| IBIS file stm32h523_533_lqfp48.ibs
[IBIS ver] 4.2
[File name] stm32h523_533_lqfp48.ibs
[File Rev] 0.2
[Date] 07-05-2024
[Source] Data Created at STMicroelectronics
[Notes]  File originated from ELDO simulations.
[Disclaimer]  This information is for modeling purpose only and is
   not guaranteed. The information is subject to change without
   notice.
[Copyright] Copyright 2024 STMicroelectronics Inc.
|   Component stm32h523_533_lqfp48
[Component] stm32h523_533_lqfp48
[Manufacturer] STMicroelectronics
[Package]
| variable   typ   min   max
R_pkg  0  NA  NA
L_pkg  0  NA  NA
C_pkg  0  NA  NA
[Pin]   signal_name   model_name
1  VBAT  power
2  PC13  io8_ft_i3c_spi_v33
3  PC14-OSC32_IN  io_ft_tamp
4  PC15-OSC32_OUT  io_ft_tamp
5  PH0-OSC_IN  io8_ft_i3c_spi
6  PH1-OSC_OUT  io8_ft_i3c_spi
7  NRST  ioreset_ft_v33
8  VSSA  nc
9  VDDA  nc
10  PA0  io8_ft_spi
11  PA1  io8_ft_spi_tamp
12  PA2  io8_ft_spi
13  PA3  io8_ft_spi
14  PA4  io8_ft_spi
15  PA5  io8_ft_spi
16  PA6  io8_ft_spi
17  PA7  io8_ft_spi
18  PB0  io8_ft_spi
19  PB1  io8_ft_spi
20  PB2  io8_ft_i3c_spi
21  PB10  io8_ft_i3c_spi
22  VCAP  nc
23  VSS  gnd
24  VDD  power
25  PB12  io8_ft_i3c_spi
26  PB13  nc
27  PB14  nc
28  PB15  io8_ft_spi
29  PA8  io8_ft_i3c_spi
30  PA9  io8_ft_i3c_spi
31  PA10  io8_ft_i3c_spi
32  PA11  io8usb_ft_i3c_spi_phy
33  PA12  io8usb_ft_i3c_spi_phy
34  PA13  io8_ft_i3c_spi
35  VSS  gnd
36  VDD  power
37  PA14  io8_ft_i3c_spi
38  PA15  io8_ft_i3c_spi
39  PB3  io8_ft_i3c_spi
40  PB4  io8_ft_i3c_spi
41  PB5  io8_ft_i3c_spi
42  PB6  io8_ft_i3c_spi
43  PB7  io8_ft_i3c_spi
44  BOOT0  vpphv
45  PB8  io8_ft_i3c_spi
46  VCAP  nc
47  VSS  gnd
48  VDD  power
[Package Model]   478-lqfp-7x7-48-240315
[Pin Mapping]   pulldown_ref   pullup_ref   | Comment
1  nc  vsw
2  gndio  vddio  | Depending on IO usage
| 2  gndio  vsw  | Depending on IO usage
3  gndio  vddio  | Depending on IO usage
| 3  gndio  vsw  | Depending on IO usage
4  gndio  vddio  | Depending on IO usage
| 4  gndio  vsw  | Depending on IO usage
5  gndio  vddio
6  gndio  vddio
7  gndio  vddio
8  nc  nc
9  nc  nc
10  gndio  vddio
11  gndio  vddio
12  gndio  vddio
13  gndio  vddio
14  gndio  vddio
15  gndio  vddio
16  gndio  vddio
17  gndio  vddio
18  gndio  vddio
19  gndio  vddio
20  gndio  vddio
21  gndio  vddio
22  nc  nc
23  gndio  nc
24  nc  vddio
25  gndio  vddio
26  nc  nc
27  nc  nc
28  gndio  vddio
29  gndio  vddio
30  gndio  vddio
31  gndio  vddio
32  gndio  vddusb  | Depending on IO usage
| 32  gndio  vddio  | Depending on IO usage
33  gndio  vddusb  | Depending on IO usage
| 33  gndio  vddio  | Depending on IO usage
34  gndio  vddio
35  gndio  nc
36  nc  vddusb
37  gndio  vddio
38  gndio  vddio
39  gndio  vddio
40  gndio  vddio
41  gndio  vddio
42  gndio  vddio
43  gndio  vddio
44  gndio  vddio
45  gndio  vddio
46  nc  nc
47  gndio  nc
48  nc  vddio
|[Diff Pin]  inv_pin  vdiff  tdelay_typ  tdelay_min  tdelay_max
|33  32  NA  NA  NA  NA
[Model Selector] io8_ft_i3c_spi
io8_ft_spi_ls_1v2 "GPIO SPI - 5V tolerant - low speed - 1.2V range"
io8_ft_spi_ls_1v8 "GPIO SPI - 5V tolerant - low speed - 1.8V range"
io8_ft_spi_ls_3v3 "GPIO SPI - 5V tolerant - low speed - 3.3V range"
io8_ft_spi_ms_1v2 "GPIO SPI - 5V tolerant - med speed - 1.2V range"
io8_ft_spi_ms_1v8 "GPIO SPI - 5V tolerant - med speed - 1.8V range"
io8_ft_spi_ms_3v3 "GPIO SPI - 5V tolerant - med speed - 3.3V range"
io8_ft_spi_fs_1v2 "GPIO SPI - 5V tolerant - fast speed - 1.2V range"
io8_ft_spi_fs_1v8 "GPIO SPI - 5V tolerant - fast speed - 1.8V range"
io8_ft_spi_fs_3v3 "GPIO SPI - 5V tolerant - fast speed - 3.3V range"
io8_ft_spi_hs_1v2 "GPIO SPI - 5V tolerant - high speed - 1.2V range"
io8_ft_spi_hs_1v8 "GPIO SPI - 5V tolerant - high speed - 1.8V range"
io8_ft_spi_hs_3v3 "GPIO SPI - 5V tolerant - high speed - 3.3V range"
io8_ft_hslv_spi_ls_1v2 "GPIO SPI low volt opt - 5V tolerant - low speed - 1.2V range"
io8_ft_hslv_spi_ls_1v8 "GPIO SPI low volt opt - 5V tolerant - low speed - 1.8V range"
io8_ft_hslv_spi_ls_2v5 "GPIO SPI low volt opt - 5V tolerant - low speed - 2.5V range"
io8_ft_hslv_spi_ms_1v2 "GPIO SPI low volt opt - 5V tolerant - med speed - 1.2V range"
io8_ft_hslv_spi_ms_1v8 "GPIO SPI low volt opt - 5V tolerant - med speed - 1.8V range"
io8_ft_hslv_spi_ms_2v5 "GPIO SPI low volt opt - 5V tolerant - med speed - 2.5V range"
io8_ft_hslv_spi_fs_1v2 "GPIO SPI low volt opt - 5V tolerant - fast speed - 1.2V range"
io8_ft_hslv_spi_fs_1v8 "GPIO SPI low volt opt - 5V tolerant - fast speed - 1.8V range"
io8_ft_hslv_spi_fs_2v5 "GPIO SPI low volt opt - 5V tolerant - fast speed - 2.5V range"
io8_ft_hslv_spi_hs_1v2 "GPIO SPI low volt opt - 5V tolerant - high speed - 1.2V range"
io8_ft_hslv_spi_hs_1v8 "GPIO SPI low volt opt - 5V tolerant - high speed - 1.8V range"
io8_ft_hslv_spi_hs_2v5 "GPIO SPI low volt opt - 5V tolerant - high speed - 2.5V range"
io8_ft_i3c_spi_ls_1v2 "GPIO SPI with I3C open-drain - 5V tolerant - low speed - 1.2V range"
io8_ft_i3c_spi_ls_1v8 "GPIO SPI with I3C open-drain - 5V tolerant - low speed - 1.8V range"
io8_ft_i3c_spi_ls_3v3 "GPIO SPI with I3C open-drain - 5V tolerant - low speed - 3.3V range"
io8_ft_i3c_spi_ms_1v2 "GPIO SPI with I3C open-drain - 5V tolerant - med speed - 1.2V range"
io8_ft_i3c_spi_ms_1v8 "GPIO SPI with I3C open-drain - 5V tolerant - med speed - 1.8V range"
io8_ft_i3c_spi_ms_3v3 "GPIO SPI with I3C open-drain - 5V tolerant - med speed - 3.3V range"
io8_ft_i3c_spi_fs_1v2 "GPIO SPI with I3C open-drain - 5V tolerant - fast speed - 1.2V range"
io8_ft_i3c_spi_fs_1v8 "GPIO SPI with I3C open-drain - 5V tolerant - fast speed - 1.8V range"
io8_ft_i3c_spi_fs_3v3 "GPIO SPI with I3C open-drain - 5V tolerant - fast speed - 3.3V range"
io8_ft_i3c_spi_hs_1v2 "GPIO SPI with I3C open-drain - 5V tolerant - high speed - 1.2V range"
io8_ft_i3c_spi_hs_1v8 "GPIO SPI with I3C open-drain - 5V tolerant - high speed - 1.8V range"
io8_ft_i3c_spi_hs_3v3 "GPIO SPI with I3C open-drain - 5V tolerant - high speed - 3.3V range"
io8_ft_hslv_i3c_spi_ls_1v2 "GPIO SPI low volt opt with I3C open-drain - 5V tolerant - low speed - 1.2V range"
io8_ft_hslv_i3c_spi_ls_1v8 "GPIO SPI low volt opt with I3C open-drain - 5V tolerant - low speed - 1.8V range"
io8_ft_hslv_i3c_spi_ls_2v5 "GPIO SPI low volt opt with I3C open-drain - 5V tolerant - low speed - 2.5V range"
io8_ft_hslv_i3c_spi_ms_1v2 "GPIO SPI low volt opt with I3C open-drain - 5V tolerant - med speed - 1.2V range"
io8_ft_hslv_i3c_spi_ms_1v8 "GPIO SPI low volt opt with I3C open-drain - 5V tolerant - med speed - 1.8V range"
io8_ft_hslv_i3c_spi_ms_2v5 "GPIO SPI low volt opt with I3C open-drain - 5V tolerant - med speed - 2.5V range"
io8_ft_hslv_i3c_spi_fs_1v2 "GPIO SPI low volt opt with I3C open-drain - 5V tolerant - fast speed - 1.2V range"
io8_ft_hslv_i3c_spi_fs_1v8 "GPIO SPI low volt opt with I3C open-drain - 5V tolerant - fast speed - 1.8V range"
io8_ft_hslv_i3c_spi_fs_2v5 "GPIO SPI low volt opt with I3C open-drain - 5V tolerant - fast speed - 2.5V range"
io8_ft_hslv_i3c_spi_hs_1v2 "GPIO SPI low volt opt with I3C open-drain - 5V tolerant - high speed - 1.2V range"
io8_ft_hslv_i3c_spi_hs_1v8 "GPIO SPI low volt opt with I3C open-drain - 5V tolerant - high speed - 1.8V range"
io8_ft_hslv_i3c_spi_hs_2v5 "GPIO SPI low volt opt with I3C open-drain - 5V tolerant - high speed - 2.5V range"
io8_ft_i3c_fmp_spi_3v3 "GPIO SPI with I3C fm+ open-drain - 5V tolerant - 3.3V range"
io8_ft_i3c_fmp_spi_1v8 "GPIO SPI with I3C fm+ open-drain - 5V tolerant - 1.8V range"
io8_ft_i3c_fmp_spi_1v2 "GPIO SPI with I3C fm+ open-drain - 5V tolerant - 1.2V range"
[Model Selector] io8_ft_i3c_spi_v33
io8_ft_spi_v33_ls_1v2 ""GPIO SPI V33 - 5V tolerant - low speed - 1.2V range"
io8_ft_spi_v33_ls_1v8 ""GPIO SPI V33 - 5V tolerant - low speed - 1.8V range"
io8_ft_spi_v33_ls_3v3 ""GPIO SPI V33 - 5V tolerant - low speed - 3.3V range"
io8_ft_spi_v33_ms_1v2 ""GPIO SPI V33 - 5V tolerant - med speed - 1.2V range"
io8_ft_spi_v33_ms_1v8 ""GPIO SPI V33 - 5V tolerant - med speed - 1.8V range"
io8_ft_spi_v33_ms_3v3 ""GPIO SPI V33 - 5V tolerant - med speed - 3.3V range"
io8_ft_spi_v33_fs_1v2 ""GPIO SPI V33 - 5V tolerant - fast speed - 1.2V range
io8_ft_spi_v33_fs_1v8 ""GPIO SPI V33 - 5V tolerant - fast speed - 1.8V range
io8_ft_spi_v33_fs_3v3 ""GPIO SPI V33 - 5V tolerant - fast speed - 3.3V range
io8_ft_spi_v33_hs_1v2 ""GPIO SPI V33 - 5V tolerant - high speed - 1.2V range
io8_ft_spi_v33_hs_1v8 ""GPIO SPI V33 - 5V tolerant - high speed - 1.8V range
io8_ft_spi_v33_hs_3v3 ""GPIO SPI V33 - 5V tolerant - high speed - 3.3V range
io8_ft_hslv_spi_v33_ls_1v2 "GPIO SPI V33 low volt opt - 5V tolerant - low speed - 1.2V range""
io8_ft_hslv_spi_v33_ls_1v8 "GPIO SPI V33 low volt opt - 5V tolerant - low speed - 1.8V range""
io8_ft_hslv_spi_v33_ls_2v5 "GPIO SPI V33 low volt opt - 5V tolerant - low speed - 2.5V range""
io8_ft_hslv_spi_v33_ms_1v2 "GPIO SPI V33 low volt opt - 5V tolerant - med speed - 1.2V range""
io8_ft_hslv_spi_v33_ms_1v8 "GPIO SPI V33 low volt opt - 5V tolerant - med speed - 1.8V range""
io8_ft_hslv_spi_v33_ms_2v5 "GPIO SPI V33 low volt opt - 5V tolerant - med speed - 2.5V range""
io8_ft_hslv_spi_v33_fs_1v2 "GPIO SPI V33 low volt opt - 5V tolerant - fast speed - 1.2V range"
io8_ft_hslv_spi_v33_fs_1v8 "GPIO SPI V33 low volt opt - 5V tolerant - fast speed - 1.8V range"
io8_ft_hslv_spi_v33_fs_2v5 "GPIO SPI V33 low volt opt - 5V tolerant - fast speed - 2.5V range"
io8_ft_hslv_spi_v33_hs_1v2 "GPIO SPI V33 low volt opt - 5V tolerant - high speed - 1.2V range"
io8_ft_hslv_spi_v33_hs_1v8 "GPIO SPI V33 low volt opt - 5V tolerant - high speed - 1.8V range"
io8_ft_hslv_spi_v33_hs_2v5 "GPIO SPI V33 low volt opt - 5V tolerant - high speed - 2.5V range"
io8_ft_i3c_spi_v33_ls_1v2 "GPIO SPI V33 with I3C open-drain - 5V tolerant - low speed - 1.2V range"
io8_ft_i3c_spi_v33_ls_1v8 "GPIO SPI V33 with I3C open-drain - 5V tolerant - low speed - 1.8V range"
io8_ft_i3c_spi_v33_ls_3v3 "GPIO SPI V33 with I3C open-drain - 5V tolerant - low speed - 3.3V range"
io8_ft_i3c_spi_v33_ms_1v2 "GPIO SPI V33 with I3C open-drain - 5V tolerant - med speed - 1.2V range"
io8_ft_i3c_spi_v33_ms_1v8 "GPIO SPI V33 with I3C open-drain - 5V tolerant - med speed - 1.8V range"
io8_ft_i3c_spi_v33_ms_3v3 "GPIO SPI V33 with I3C open-drain - 5V tolerant - med speed - 3.3V range"
io8_ft_i3c_spi_v33_fs_1v2 "GPIO SPI V33 with I3C open-drain - 5V tolerant - fast speed - 1.2V range"
io8_ft_i3c_spi_v33_fs_1v8 "GPIO SPI V33 with I3C open-drain - 5V tolerant - fast speed - 1.8V range"
io8_ft_i3c_spi_v33_fs_3v3 "GPIO SPI V33 with I3C open-drain - 5V tolerant - fast speed - 3.3V range"
io8_ft_i3c_spi_v33_hs_1v2 "GPIO SPI V33 with I3C open-drain - 5V tolerant - high speed - 1.2V range"
io8_ft_i3c_spi_v33_hs_1v8 "GPIO SPI V33 with I3C open-drain - 5V tolerant - high speed - 1.8V range"
io8_ft_i3c_spi_v33_hs_3v3 "GPIO SPI V33 with I3C open-drain - 5V tolerant - high speed - 3.3V range"
io8_ft_hslv_i3c_spi_v33_ls_1v2 "GPIO SPI V33 low volt opt with I3C open-drain - 5V tolerant - low speed - 1.2V range"
io8_ft_hslv_i3c_spi_v33_ls_1v8 "GPIO SPI V33 low volt opt with I3C open-drain - 5V tolerant - low speed - 1.8V range"
io8_ft_hslv_i3c_spi_v33_ls_2v5 "GPIO SPI V33 low volt opt with I3C open-drain - 5V tolerant - low speed - 2.5V range"
io8_ft_hslv_i3c_spi_v33_ms_1v2 "GPIO SPI V33 low volt opt with I3C open-drain - 5V tolerant - med speed - 1.2V range"
io8_ft_hslv_i3c_spi_v33_ms_1v8 "GPIO SPI V33 low volt opt with I3C open-drain - 5V tolerant - med speed - 1.8V range"
io8_ft_hslv_i3c_spi_v33_ms_2v5 "GPIO SPI V33 low volt opt with I3C open-drain - 5V tolerant - med speed - 2.5V range"
io8_ft_hslv_i3c_spi_v33_fs_1v2 "GPIO SPI V33 low volt opt with I3C open-drain - 5V tolerant - fast speed - 1.2V range"
io8_ft_hslv_i3c_spi_v33_fs_1v8 "GPIO SPI V33 low volt opt with I3C open-drain - 5V tolerant - fast speed - 1.8V range"
io8_ft_hslv_i3c_spi_v33_fs_2v5 "GPIO SPI V33 low volt opt with I3C open-drain - 5V tolerant - fast speed - 2.5V range"
io8_ft_hslv_i3c_spi_v33_hs_1v2 "GPIO SPI V33 low volt opt with I3C open-drain - 5V tolerant - high speed - 1.2V range"
io8_ft_hslv_i3c_spi_v33_hs_1v8 "GPIO SPI V33 low volt opt with I3C open-drain - 5V tolerant - high speed - 1.8V range"
io8_ft_hslv_i3c_spi_v33_hs_2v5 "GPIO SPI V33 low volt opt with I3C open-drain - 5V tolerant - high speed - 2.5V range"
io8_ft_i3c_fmp_spi_v33_3v3 "GPIO SPI V33 with I3C fm+ open-drain - 5V tolerant - 3.3V range"
io8_ft_i3c_fmp_spi_v33_1v8 "GPIO SPI V33 with I3C fm+ open-drain - 5V tolerant - 1.8V range"
io8_ft_i3c_fmp_spi_v33_1v2 "GPIO SPI V33 with I3C fm+ open-drain - 5V tolerant - 1.2V range"
[Model Selector] io8_ft_spi
io8_ft_spi_ls_1v2 "GPIO SPI - 5V tolerant - low speed - 1.2V range"
io8_ft_spi_ls_1v8 "GPIO SPI - 5V tolerant - low speed - 1.8V range"
io8_ft_spi_ls_3v3 "GPIO SPI - 5V tolerant - low speed - 3.3V range"
io8_ft_spi_ms_1v2 "GPIO SPI- 5V tolerant - med speed - 1.2V range"
io8_ft_spi_ms_1v8 "GPIO SPI- 5V tolerant - med speed - 1.8V range"
io8_ft_spi_ms_3v3 "GPIO SPI- 5V tolerant - med speed - 3.3V range"
io8_ft_spi_fs_1v2 "GPIO SPI- 5V tolerant - fast speed - 1.2V range"
io8_ft_spi_fs_1v8 "GPIO SPI- 5V tolerant - fast speed - 1.8V range"
io8_ft_spi_fs_3v3 "GPIO SPI- 5V tolerant - fast speed - 3.3V range"
io8_ft_spi_hs_1v2 "GPIO SPI- 5V tolerant - high speed - 1.2V range"
io8_ft_spi_hs_1v8 "GPIO SPI- 5V tolerant - high speed - 1.8V range"
io8_ft_spi_hs_3v3 "GPIO SPI- 5V tolerant - high speed - 3.3V range"
io8_ft_hslv_spi_ls_1v2 "GPIO SPI low volt opt - 5V tolerant - low speed - 1.2V range"
io8_ft_hslv_spi_ls_1v8 "GPIO SPI low volt opt - 5V tolerant - low speed - 1.8V range"
io8_ft_hslv_spi_ls_2v5 "GPIO SPI low volt opt - 5V tolerant - low speed - 2.5V range"
io8_ft_hslv_spi_ms_1v2 "GPIO SPI low volt opt - 5V tolerant - med speed - 1.2V range"
io8_ft_hslv_spi_ms_1v8 "GPIO SPI low volt opt - 5V tolerant - med speed - 1.8V range"
io8_ft_hslv_spi_ms_2v5 "GPIO SPI low volt opt - 5V tolerant - med speed - 2.5V range"
io8_ft_hslv_spi_fs_1v2 "GPIO SPI low volt opt - 5V tolerant - fast speed - 1.2V range"
io8_ft_hslv_spi_fs_1v8 "GPIO SPI low volt opt - 5V tolerant - fast speed - 1.8V range"
io8_ft_hslv_spi_fs_2v5 "GPIO SPI low volt opt - 5V tolerant - fast speed - 2.5V range"
io8_ft_hslv_spi_hs_1v2 "GPIO SPI low volt opt - 5V tolerant - high speed - 1.2V range"
io8_ft_hslv_spi_hs_1v8 "GPIO SPI low volt opt - 5V tolerant - high speed - 1.8V range"
io8_ft_hslv_spi_hs_2v5 "GPIO SPI low volt opt - 5V tolerant - high speed - 2.5V range"
[Model Selector] io8_ft_spi_tamp
io8_ft_spi_ls_1v2 "GPIO SPI - 5V tolerant - low speed - 1.2V range"
io8_ft_spi_ls_1v8 "GPIO SPI - 5V tolerant - low speed - 1.8V range"
io8_ft_spi_ls_3v3 "GPIO SPI- 5V tolerant - low speed - 3.3V range"
io8_ft_spi_ms_1v2 "GPIO SPI - 5V tolerant - med speed - 1.2V range"
io8_ft_spi_ms_1v8 "GPIO SPI - 5V tolerant - med speed - 1.8V range"
io8_ft_spi_ms_3v3 "GPIO SPI - 5V tolerant - med speed - 3.3V range"
io8_ft_spi_fs_1v2 "GPIO SPI - 5V tolerant - fast speed - 1.2V range"
io8_ft_spi_fs_1v8 "GPIO SPI - 5V tolerant - fast speed - 1.8V range"
io8_ft_spi_fs_3v3 "GPIO SPI - 5V tolerant - fast speed - 3.3V range"
io8_ft_spi_hs_1v2 "GPIO SPI - 5V tolerant - high speed - 1.2V range"
io8_ft_spi_hs_1v8 "GPIO SPI - 5V tolerant - high speed - 1.8V range"
io8_ft_spi_hs_3v3 "GPIO SPI - 5V tolerant - high speed - 3.3V range"
io8_ft_hslv_spi_ls_1v2 "GPIO SPI low volt opt - 5V tolerant - low speed - 1.2V range"
io8_ft_hslv_spi_ls_1v8 "GPIO SPI low volt opt - 5V tolerant - low speed - 1.8V range"
io8_ft_hslv_spi_ls_2v5 "GPIO SPI low volt opt - 5V tolerant - low speed - 2.5V range"
io8_ft_hslv_spi_ms_1v2 "GPIO SPI low volt opt - 5V tolerant - med speed - 1.2V range"
io8_ft_hslv_spi_ms_1v8 "GPIO SPI low volt opt - 5V tolerant - med speed - 1.8V range"
io8_ft_hslv_spi_ms_2v5 "GPIO SPI low volt opt - 5V tolerant - med speed - 2.5V range"
io8_ft_hslv_spi_fs_1v2 "GPIO SPI low volt opt - 5V tolerant - fast speed - 1.2V range"
io8_ft_hslv_spi_fs_1v8 "GPIO SPI low volt opt - 5V tolerant - fast speed - 1.8V range"
io8_ft_hslv_spi_fs_2v5 "GPIO SPI low volt opt - 5V tolerant - fast speed - 2.5V range"
io8_ft_hslv_spi_hs_1v2 "GPIO SPI low volt opt - 5V tolerant - high speed - 1.2V range"
io8_ft_hslv_spi_hs_1v8 "GPIO SPI low volt opt - 5V tolerant - high speed - 1.8V range"
io8_ft_hslv_spi_hs_2v5 "GPIO SPI low volt opt - 5V tolerant - high speed - 2.5V range
io8_ft_tamp_v33_1v2 "IO tamper - 5V tolerant - 1.2V range"
io8_ft_tamp_v33_1v8 "IO tamper - 5V tolerant - 1.8V range"
io8_ft_tamp_v33_3v3 "IO tamper - 5V tolerant - 3.3V range"
[Model Selector] io8usb_ft_i3c_spi_phy
io8_ft_spi_ls_1v2 "GPIO SPI - 5V tolerant - low speed - 1.2V range"
io8_ft_spi_ls_1v8 "GPIO SPI - 5V tolerant - low speed - 1.8V range"
io8_ft_spi_ls_3v3 "GPIO SPI - 5V tolerant - low speed - 3.3V range"
io8_ft_spi_ms_1v2 "GPIO SPI - 5V tolerant - med speed - 1.2V range"
io8_ft_spi_ms_1v8 "GPIO SPI - 5V tolerant - med speed - 1.8V range"
io8_ft_spi_ms_3v3 "GPIO SPI - 5V tolerant - med speed - 3.3V range"
io8_ft_spi_fs_1v2 "GPIO SPI - 5V tolerant - fast speed - 1.2V range"
io8_ft_spi_fs_1v8 "GPIO SPI - 5V tolerant - fast speed - 1.8V range"
io8_ft_spi_fs_3v3 "GPIO SPI - 5V tolerant - fast speed - 3.3V range"
io8_ft_spi_hs_1v2 "GPIO SPI - 5V tolerant - high speed - 1.2V range"
io8_ft_spi_hs_1v8 "GPIO SPI - 5V tolerant - high speed - 1.8V range"
io8_ft_spi_hs_3v3 "GPIO SPI - 5V tolerant - high speed - 3.3V range"
io8_ft_hslv_spi_ls_1v2 "GPIO SPI low volt opt - 5V tolerant - low speed - 1.2V range"
io8_ft_hslv_spi_ls_1v8 "GPIO SPI low volt opt - 5V tolerant - low speed - 1.8V range"
io8_ft_hslv_spi_ls_2v5 "GPIO SPI low volt opt - 5V tolerant - low speed - 2.5V range"
io8_ft_hslv_spi_ms_1v2 "GPIO SPI low volt opt - 5V tolerant - med speed - 1.2V range"
io8_ft_hslv_spi_ms_1v8 "GPIO SPI low volt opt - 5V tolerant - med speed - 1.8V range"
io8_ft_hslv_spi_ms_2v5 "GPIO SPI low volt opt - 5V tolerant - med speed - 2.5V range"
io8_ft_hslv_spi_fs_1v2 "GPIO SPI low volt opt - 5V tolerant - fast speed - 1.2V range"
io8_ft_hslv_spi_fs_1v8 "GPIO SPI low volt opt - 5V tolerant - fast speed - 1.8V range"
io8_ft_hslv_spi_fs_2v5 "GPIO SPI low volt opt - 5V tolerant - fast speed - 2.5V range"
io8_ft_hslv_spi_hs_1v2 "GPIO SPI low volt opt - 5V tolerant - high speed - 1.2V range"
io8_ft_hslv_spi_hs_1v8 "GPIO SPI low volt opt - 5V tolerant - high speed - 1.8V range"
io8_ft_hslv_spi_hs_2v5 "GPIO SPI low volt opt - 5V tolerant - high speed - 2.5V range"
io8_ft_i3c_spi_ls_1v2 "GPIO SPI  with I3C open-drain - 5V tolerant - low speed - 1.2V range"
io8_ft_i3c_spi_ls_1v8 "GPIO SPI  with I3C open-drain - 5V tolerant - low speed - 1.8V range"
io8_ft_i3c_spi_ls_3v3 "GPIO SPI  with I3C open-drain - 5V tolerant - low speed - 3.3V range"
io8_ft_i3c_spi_ms_1v2 "GPIO SPI  with I3C open-drain - 5V tolerant - med speed - 1.2V range"
io8_ft_i3c_spi_ms_1v8 "GPIO SPI  with I3C open-drain - 5V tolerant - med speed - 1.8V range"
io8_ft_i3c_spi_ms_3v3 "GPIO SPI  with I3C open-drain - 5V tolerant - med speed - 3.3V range"
io8_ft_i3c_spi_fs_1v2 "GPIO SPI  with I3C open-drain - 5V tolerant - fast speed - 1.2V range"
io8_ft_i3c_spi_fs_1v8 "GPIO SPI  with I3C open-drain - 5V tolerant - fast speed - 1.8V range"
io8_ft_i3c_spi_fs_3v3 "GPIO SPI  with I3C open-drain - 5V tolerant - fast speed - 3.3V range"
io8_ft_i3c_spi_hs_1v2 "GPIO SPI  with I3C open-drain - 5V tolerant - high speed - 1.2V range"
io8_ft_i3c_spi_hs_1v8 "GPIO SPI  with I3C open-drain - 5V tolerant - high speed - 1.8V range"
io8_ft_i3c_spi_hs_3v3 "GPIO SPI  with I3C open-drain - 5V tolerant - high speed - 3.3V range"
io8_ft_hslv_i3c_spi_ls_1v2 "GPIO SPI  low volt opt with I3C open-drain - 5V tolerant - low speed - 1.2V range"
io8_ft_hslv_i3c_spi_ls_1v8 "GPIO SPI  low volt opt with I3C open-drain - 5V tolerant - low speed - 1.8V range"
io8_ft_hslv_i3c_spi_ls_2v5 "GPIO SPI  low volt opt with I3C open-drain - 5V tolerant - low speed - 2.5V range"
io8_ft_hslv_i3c_spi_ms_1v2 "GPIO SPI  low volt opt with I3C open-drain - 5V tolerant - med speed - 1.2V range"
io8_ft_hslv_i3c_spi_ms_1v8 "GPIO SPI  low volt opt with I3C open-drain - 5V tolerant - med speed - 1.8V range"
io8_ft_hslv_i3c_spi_ms_2v5 "GPIO SPI  low volt opt with I3C open-drain - 5V tolerant - med speed - 2.5V range"
io8_ft_hslv_i3c_spi_fs_1v2 "GPIO SPI  low volt opt with I3C open-drain - 5V tolerant - fast speed - 1.2V range"
io8_ft_hslv_i3c_spi_fs_1v8 "GPIO SPI  low volt opt with I3C open-drain - 5V tolerant - fast speed - 1.8V range"
io8_ft_hslv_i3c_spi_fs_2v5 "GPIO SPI  low volt opt with I3C open-drain - 5V tolerant - fast speed - 2.5V range"
io8_ft_hslv_i3c_spi_hs_1v2 "GPIO SPI  low volt opt with I3C open-drain - 5V tolerant - high speed - 1.2V range"
io8_ft_hslv_i3c_spi_hs_1v8 "GPIO SPI  low volt opt with I3C open-drain - 5V tolerant - high speed - 1.8V range"
io8_ft_hslv_i3c_spi_hs_2v5 "GPIO SPI  low volt opt with I3C open-drain - 5V tolerant - high speed - 2.5V range"
io8_ft_i3c_fmp_spi_3v3 "GPIO SPI  with I3C fm+ open-drain - 5V tolerant - 3.3V range"
io8_ft_i3c_fmp_spi_1v8 "GPIO SPI  with I3C fm+ open-drain - 5V tolerant - 1.8V range"
io8_ft_i3c_fmp_spi_1v2 "GPIO SPI  with I3C fm+ open-drain - 5V tolerant - 1.2V range"
io8usb_ft_phy_ls_2v5 "USB PHY - 5V tolerant - low speed - 2.5V range"
io8usb_ft_phy_ls_3v3 "USB PHY - 5V tolerant - low speed - 3.3V range
io8usb_ft_phy_fs_2v5 "USB PHY - 5V tolerant - fast speed - 2.5V range"
io8usb_ft_phy_fs_3v3 "USB PHY - 5V tolerant - fast speed - 3.3V range"
[Model Selector] io_ft_tamp
io_ft_tamp_3v3 "IO tamper - 5V tolerant - 3.3V range"
io_ft_tamp_1v8 "IO tamper - 5V tolerant - 1.8V range"
io_ft_tamp_1v2 "IO tamper - 5V tolerant - 1.2V range"
[Model Selector] ioreset_ft_v33
ioreset_ft_v33_1v2 "Reset PAD. 5V tolerant. 1.2V range"
ioreset_ft_v33_1v8 "Reset PAD. 5V tolerant. 1.8V range"
ioreset_ft_v33_3v3 "Reset PAD. 5V tolerant. 3.3V range"
[Model Selector] vpphv
vpphv_1v2 "Flash Test cell v33 = 1.2 V range"
vpphv_1v8 "Flash Test cell v33 = 1.8 V range"
vpphv_3v3 "Flash Test cell v33 = 3.3 V range"
[Define Package Model]  478-lqfp-7x7-48-240315
[Manufacturer]  Unknown
[OEM]  Unknown
[Description]  None
[Number Of Pins]  46
[Pin Numbers]
| Pin Num   Terminal Name
7 | NRST
10 | PA0
31 | PA10
32 | PA11
33 | PA12
34 | PA13
37 | PA14
38 | PA15
11 | PA1
12 | PA2
13 | PA3
14 | PA4
15 | PA5
16 | PA6
17 | PA7
29 | PA8
30 | PA9
18 | PB0
21 | PB10
25 | PB12
26 | PB13
27 | PB14
28 | PB15
19 | PB1
20 | PB2
39 | PB3
40 | PB4
41 | PB5
42 | PB6
43 | PB7
45 | PB8
2 | PC13
3 | PC14-OSC32_IN
4 | PC15-OSC32_OUT
5 | PH0-OSC_IN
6 | PH1-OSC_OUT
1 | VBAT
22 | VCAP
46 | VCAP
24 | VDD
36 | VDD
48 | VDD
9 | VDDA
44 | BOOT0
23 | VSS
8 | VSSA
|[Merged Pins]  23
|35  |  VSS
|47  |  VSS
[Model Data]
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[End Model Data]
[End Package Model]
|End [Component]
| Models and submodels in the file (118): io8_ft_hslv_i3c_spi_fs_1v2 (I/O_open_drain), io8_ft_hslv_i3c_spi_fs_1v8 (I/O_open_drain), io8_ft_hslv_i3c_spi_fs_2v5 (I/O_open_drain), io8_ft_hslv_i3c_spi_hs_1v2 (I/O_open_drain), io8_ft_hslv_i3c_spi_hs_1v8 (I/O_open_drain), io8_ft_hslv_i3c_spi_hs_2v5 (I/O_open_drain), io8_ft_hslv_i3c_spi_ls_1v2 (I/O_open_drain), io8_ft_hslv_i3c_spi_ls_1v8 (I/O_open_drain), io8_ft_hslv_i3c_spi_ls_2v5 (I/O_open_drain), io8_ft_hslv_i3c_spi_ms_1v2 (I/O_open_drain), io8_ft_hslv_i3c_spi_ms_1v8 (I/O_open_drain), io8_ft_hslv_i3c_spi_ms_2v5 (I/O_open_drain), io8_ft_hslv_i3c_spi_v33_fs_1v2 (I/O_open_drain), io8_ft_hslv_i3c_spi_v33_fs_1v8 (I/O_open_drain), io8_ft_hslv_i3c_spi_v33_fs_2v5 (I/O_open_drain), io8_ft_hslv_i3c_spi_v33_hs_1v2 (I/O_open_drain), io8_ft_hslv_i3c_spi_v33_hs_1v8 (I/O_open_drain), io8_ft_hslv_i3c_spi_v33_hs_2v5 (I/O_open_drain), io8_ft_hslv_i3c_spi_v33_ls_1v2 (I/O_open_drain), io8_ft_hslv_i3c_spi_v33_ls_1v8 (I/O_open_drain), io8_ft_hslv_i3c_spi_v33_ls_2v5 (I/O_open_drain), io8_ft_hslv_i3c_spi_v33_ms_1v2 (I/O_open_drain), io8_ft_hslv_i3c_spi_v33_ms_1v8 (I/O_open_drain), io8_ft_hslv_i3c_spi_v33_ms_2v5 (I/O_open_drain), io8_ft_hslv_spi_fs_1v2 (I/O), io8_ft_hslv_spi_fs_1v8 (I/O), io8_ft_hslv_spi_fs_2v5 (I/O), io8_ft_hslv_spi_hs_1v2 (I/O), io8_ft_hslv_spi_hs_1v8 (I/O), io8_ft_hslv_spi_hs_2v5 (I/O), io8_ft_hslv_spi_ls_1v2 (I/O), io8_ft_hslv_spi_ls_1v8 (I/O), io8_ft_hslv_spi_ls_2v5 (I/O), io8_ft_hslv_spi_ms_1v2 (I/O), io8_ft_hslv_spi_ms_1v8 (I/O), io8_ft_hslv_spi_ms_2v5 (I/O), io8_ft_hslv_spi_v33_fs_1v2 (I/O), io8_ft_hslv_spi_v33_fs_1v8 (I/O), io8_ft_hslv_spi_v33_fs_2v5 (I/O), io8_ft_hslv_spi_v33_hs_1v2 (I/O), io8_ft_hslv_spi_v33_hs_1v8 (I/O), io8_ft_hslv_spi_v33_hs_2v5 (I/O), io8_ft_hslv_spi_v33_ls_1v2 (I/O), io8_ft_hslv_spi_v33_ls_1v8 (I/O), io8_ft_hslv_spi_v33_ls_2v5 (I/O), io8_ft_hslv_spi_v33_ms_1v2 (I/O), io8_ft_hslv_spi_v33_ms_1v8 (I/O), io8_ft_hslv_spi_v33_ms_2v5 (I/O), io8_ft_i3c_fmp_spi_1v2 (I/O_open_drain), io8_ft_i3c_fmp_spi_1v8 (I/O_open_drain), io8_ft_i3c_fmp_spi_3v3 (I/O_open_drain), io8_ft_i3c_fmp_spi_v33_1v2 (I/O_open_drain), io8_ft_i3c_fmp_spi_v33_1v8 (I/O_open_drain), io8_ft_i3c_fmp_spi_v33_3v3 (I/O_open_drain), io8_ft_i3c_spi_fs_1v2 (I/O_open_drain), io8_ft_i3c_spi_fs_1v8 (I/O_open_drain), io8_ft_i3c_spi_fs_3v3 (I/O_open_drain), io8_ft_i3c_spi_hs_1v2 (I/O_open_drain), io8_ft_i3c_spi_hs_1v8 (I/O_open_drain), io8_ft_i3c_spi_hs_3v3 (I/O_open_drain), io8_ft_i3c_spi_ls_1v2 (I/O_open_drain), io8_ft_i3c_spi_ls_1v8 (I/O_open_drain), io8_ft_i3c_spi_ls_3v3 (I/O_open_drain), io8_ft_i3c_spi_ms_1v2 (I/O_open_drain), io8_ft_i3c_spi_ms_1v8 (I/O_open_drain), io8_ft_i3c_spi_ms_3v3 (I/O_open_drain), io8_ft_i3c_spi_v33_fs_1v2 (I/O_open_drain), io8_ft_i3c_spi_v33_fs_1v8 (I/O_open_drain), io8_ft_i3c_spi_v33_fs_3v3 (I/O_open_drain), io8_ft_i3c_spi_v33_hs_1v2 (I/O_open_drain), io8_ft_i3c_spi_v33_hs_1v8 (I/O_open_drain), io8_ft_i3c_spi_v33_hs_3v3 (I/O_open_drain), io8_ft_i3c_spi_v33_ls_1v2 (I/O_open_drain), io8_ft_i3c_spi_v33_ls_1v8 (I/O_open_drain), io8_ft_i3c_spi_v33_ls_3v3 (I/O_open_drain), io8_ft_i3c_spi_v33_ms_1v2 (I/O_open_drain), io8_ft_i3c_spi_v33_ms_1v8 (I/O_open_drain), io8_ft_i3c_spi_v33_ms_3v3 (I/O_open_drain), io8_ft_spi_fs_1v2 (I/O), io8_ft_spi_fs_1v8 (I/O)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
